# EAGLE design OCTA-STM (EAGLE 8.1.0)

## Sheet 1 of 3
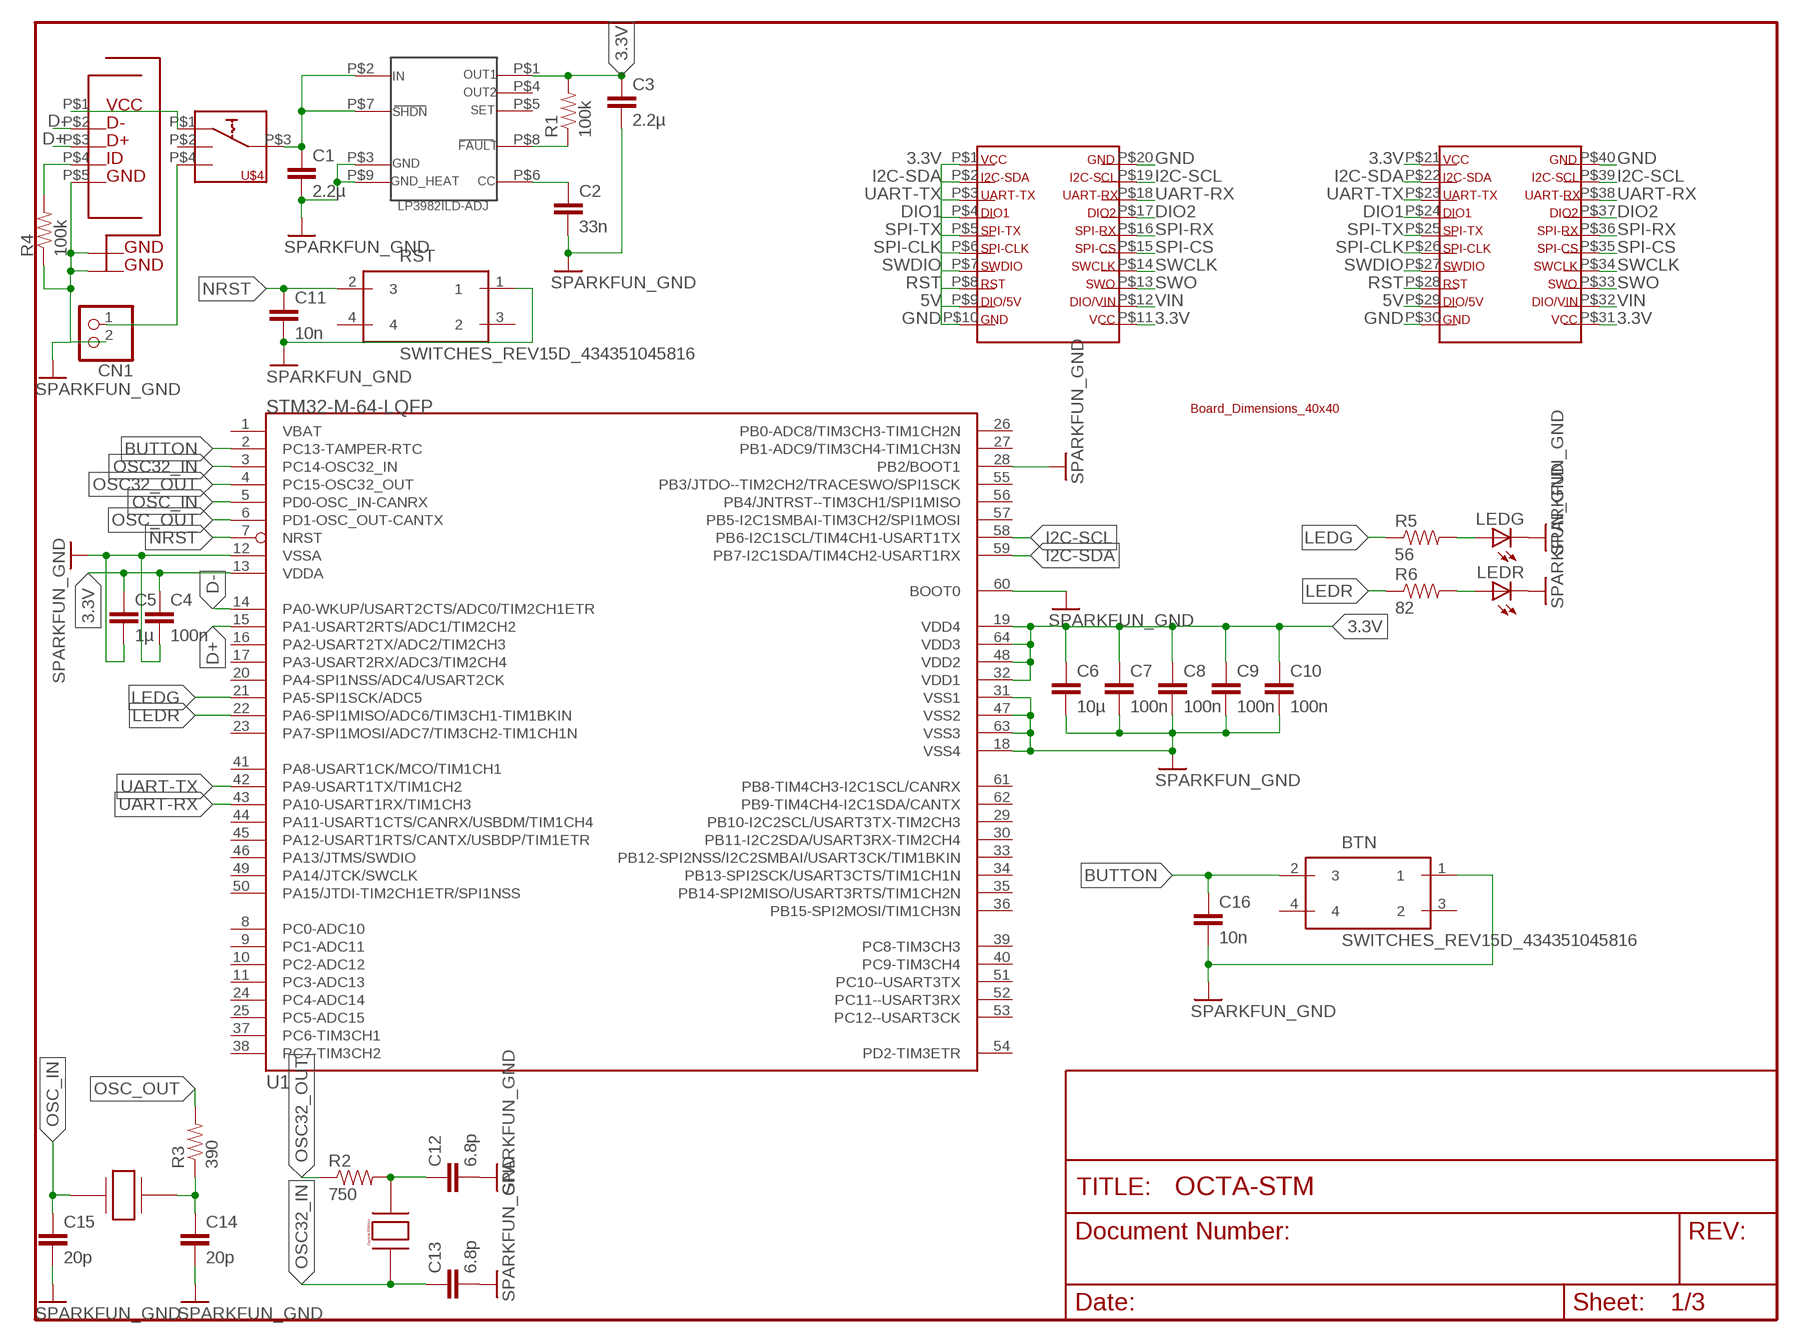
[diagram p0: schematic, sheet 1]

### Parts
8MHZ  OCTA-CORE_CRYSTAL-48MHZ  [OCTA-CORE_CRYSTAL-48MHZ]
BTN  SWITCHES_REV15D_434351045816  [SWITCHES_REV15D_434351045816]
C1  2.2µ  SPARKFUN_CAP0603-CAP  [SPARKFUN_0603-CAP]
C2  33n  SPARKFUN_CAP0603-CAP  [SPARKFUN_0603-CAP]
C3  2.2µ  SPARKFUN_CAP0603-CAP  [SPARKFUN_0603-CAP]
C4  100n  SPARKFUN_CAP0603-CAP  [SPARKFUN_0603-CAP]
C5  1µ  SPARKFUN_CAP0603-CAP  [SPARKFUN_0603-CAP]
C6  10µ  SPARKFUN_CAP0603-CAP  [SPARKFUN_0603-CAP]
C7  100n  SPARKFUN_CAP0603-CAP  [SPARKFUN_0603-CAP]
C8  100n  SPARKFUN_CAP0603-CAP  [SPARKFUN_0603-CAP]
C9  100n  SPARKFUN_CAP0603-CAP  [SPARKFUN_0603-CAP]
C10  100n  SPARKFUN_CAP0603-CAP  [SPARKFUN_0603-CAP]
C11  10n  SPARKFUN_CAP0603-CAP  [SPARKFUN_0603-CAP]
C12  6.8p  SPARKFUN_CAP0603-CAP  [SPARKFUN_0603-CAP]
C13  6.8p  SPARKFUN_CAP0603-CAP  [SPARKFUN_0603-CAP]
C14  20p  SPARKFUN_CAP0603-CAP  [SPARKFUN_0603-CAP]
C15  20p  SPARKFUN_CAP0603-CAP  [SPARKFUN_0603-CAP]
C16  10n  SPARKFUN_CAP0603-CAP  [SPARKFUN_0603-CAP]
CN1  ADAFRUIT_JST_2PIN-SMT-RA  [ADAFRUIT_JST-PH-2-SMT-RA]
LEDG  LED_LEDCHIP-LED0805  [LED_CHIP-LED0805]
LEDR  LED_LEDCHIP-LED0805  [LED_CHIP-LED0805]
R1  100k  SPARKFUN_RESISTOR0603-RES  [SPARKFUN_0603-RES]
R2  750  SPARKFUN_RESISTOR0603-RES  [SPARKFUN_0603-RES]
R3  390  SPARKFUN_RESISTOR0603-RES  [SPARKFUN_0603-RES]
R4  100k  SPARKFUN_RESISTOR0603-RES  [SPARKFUN_0603-RES]
R5  56  SPARKFUN_RESISTOR0603-RES  [SPARKFUN_0603-RES]
R6  82  SPARKFUN_RESISTOR0603-RES  [SPARKFUN_0603-RES]
RST  SWITCHES_REV15D_434351045816  [SWITCHES_REV15D_434351045816]
U1  STM32-M-64-LQFP  [LQFP64]
U$1  OCTA-CORE_MCIRO-USB2  [OCTA-CORE_MICRO-USB2]
U$2  BOARD-DIMENSIONS-40X40  [BOARD-DIMENSIONS-40X40]
U$3  DRAGAN-PERSONAL_TI-3.3V-REGULATOR  [DRAGAN-PERSONAL_TI-3.3V-REGULATOR]
U$4  OCTA-CORE_SP3T  [OCTA-CORE_SP3T]
U$5  DRAGAN-PERSONAL_CRYSTAL_32MHZ  [DRAGAN-PERSONAL_CRYSTAL_32MHZ]

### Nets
3.3V: C3.1 C4.1 C5.1 C6.1 C7.1 C8.1 C9.1 C10.1 R1.2 U1.13(VDDA) U1.19(VDD4) U1.32(VDD1) U1.48(VDD2) U1.64(VDD3) U$2.P$1 U$2.P$11 U$2.P$21 U$2.P$31 U$3.P$1 ; also sheet 2,3
5V: U$2.P$9 U$2.P$29
BUTTON: BTN.2 C16.1 U1.2(PC13-TAMPER-RTC)
D+: U1.15(PA1-USART2RTS/ADC1/TIM2CH2) U$1.P$3
D-: U1.14(PA0-WKUP/USART2CTS/ADC0/TIM2CH1ETR) U$1.P$2
DIO1: U$2.P$4 U$2.P$24
DIO2: U$2.P$17 U$2.P$37
GND: BTN.1 C1.2 C2.2 C3.2 C4.2 C5.2 C6.2 C7.2 C8.2 C9.2 C10.2 C11.2 C12.2 C13.2 C14.2 C15.2 C16.2 CN1.2 LEDG.C LEDR.C R4.1 RST.1 U1.12(VSSA) U1.18(VSS4) U1.28(PB2/BOOT1) U1.31(VSS1) U1.47(VSS2) U1.60(BOOT0) U1.63(VSS3) U$1.P$5 U$1.P$6 U$1.P$7 U$1.P$8 U$1.P$9 U$1.P$10 U$1.P$11 U$1.P$12 U$1.P$13 U$2.P$10 U$2.P$20 U$2.P$30 U$2.P$40 U$3.P$3 U$3.P$9 ; supply symbol labelled SPARKFUN_GND ; also sheet 2,3
I2C-SCL: U1.58(PB6-I2C1SCL/TIM4CH1-USART1TX) U$2.P$19 U$2.P$39 ; also sheet 2,3
I2C-SDA: U1.59(PB7-I2C1SDA/TIM4CH2-USART1RX) U$2.P$2 U$2.P$22 ; also sheet 2,3
LEDG: R5.1 U1.21(PA5-SPI1SCK/ADC5)
LEDR: R6.1 U1.22(PA6-SPI1MISO/ADC6/TIM3CH1-TIM1BKIN)
N$1: LEDG.A R5.2
N$2: CN1.1 U$4.P$4
N$3: U$1.P$1 U$4.P$1
N$4: C1.1 U$3.P$2 U$3.P$7 U$4.P$3
N$5: C2.1 U$3.P$6
N$6: C12.1 R2.2 U$5.P$2
N$7: R1.1 U$3.P$8
N$8: R4.2 U$1.P$4
N$9: 8MHZ.P$3 C14.1 R3.1
N$10: LEDR.A R6.2
NRST: C11.1 RST.2 U1.7(NRST)
OSC32_IN: C13.1 U1.3(PC14-OSC32_IN) U$5.P$3
OSC32_OUT: R2.1 U1.4(PC15-OSC32_OUT)
OSC_IN: 8MHZ.P$1 C15.1 U1.5(PD0-OSC_IN-CANRX)
OSC_OUT: R3.2 U1.6(PD1-OSC_OUT-CANTX)
RST: U$2.P$8 U$2.P$28
SPI-CLK: U$2.P$6 U$2.P$26
SPI-CS: U$2.P$15 U$2.P$35
SPI-RX: U$2.P$16 U$2.P$36
SPI-TX: U$2.P$5 U$2.P$25
SWCLK: U$2.P$14 U$2.P$34
SWDIO: U$2.P$7 U$2.P$27
SWO: U$2.P$13 U$2.P$33
UART-RX: U1.43(PA10-USART1RX/TIM1CH3) U$2.P$18 U$2.P$38
UART-TX: U1.42(PA9-USART1TX/TIM1CH2) U$2.P$3 U$2.P$23
VIN: U$2.P$12 U$2.P$32
Unconnected: 8MHZ.P$2 8MHZ.P$4 BTN.3 BTN.4 RST.3 RST.4 U1.1(VBAT) U1.8(PC0-ADC10) U1.9(PC1-ADC11) U1.10(PC2-ADC12) U1.11(PC3-ADC13) U1.16(PA2-USART2TX/ADC2/TIM2CH3) U1.17(PA3-USART2RX/ADC3/TIM2CH4) U1.20(PA4-SPI1NSS/ADC4/USART2CK) U1.23(PA7-SPI1MOSI/ADC7/TIM3CH2-TIM1CH1N) U1.24(PC4-ADC14) U1.25(PC5-ADC15) U1.26(PB0-ADC8/TIM3CH3-TIM1CH2N) U1.27(PB1-ADC9/TIM3CH4-TIM1CH3N) U1.29(PB10-I2C2SCL/USART3TX-TIM2CH3) U1.30(PB11-I2C2SDA/USART3RX-TIM2CH4) U1.33(PB12-SPI2NSS/I2C2SMBAI/USART3CK/TIM1BKIN) U1.34(PB13-SPI2SCK/USART3CTS/TIM1CH1N) U1.35(PB14-SPI2MISO/USART3RTS/TIM1CH2N) U1.36(PB15-SPI2MOSI/TIM1CH3N) U1.37(PC6-TIM3CH1) U1.38(PC7-TIM3CH2) U1.39(PC8-TIM3CH3) U1.40(PC9-TIM3CH4) U1.41(PA8-USART1CK/MCO/TIM1CH1) U1.44(PA11-USART1CTS/CANRX/USBDM/TIM1CH4) U1.45(PA12-USART1RTS/CANTX/USBDP/TIM1ETR) U1.46(PA13/JTMS/SWDIO) U1.49(PA14/JTCK/SWCLK) U1.50(PA15/JTDI-TIM2CH1ETR/SPI1NSS) U1.51(PC10--USART3TX) U1.52(PC11--USART3RX) U1.53(PC12--USART3CK) U1.54(PD2-TIM3ETR) U1.55(PB3/JTDO--TIM2CH2/TRACESWO/SPI1SCK) U1.56(PB4/JNTRST--TIM3CH1/SPI1MISO) U1.57(PB5-I2C1SMBAI-TIM3CH2/SPI1MOSI) U1.61(PB8-TIM4CH3-I2C1SCL/CANRX) U1.62(PB9-TIM4CH4-I2C1SDA/CANTX) U$3.P$4 U$3.P$5 U$4.P$2

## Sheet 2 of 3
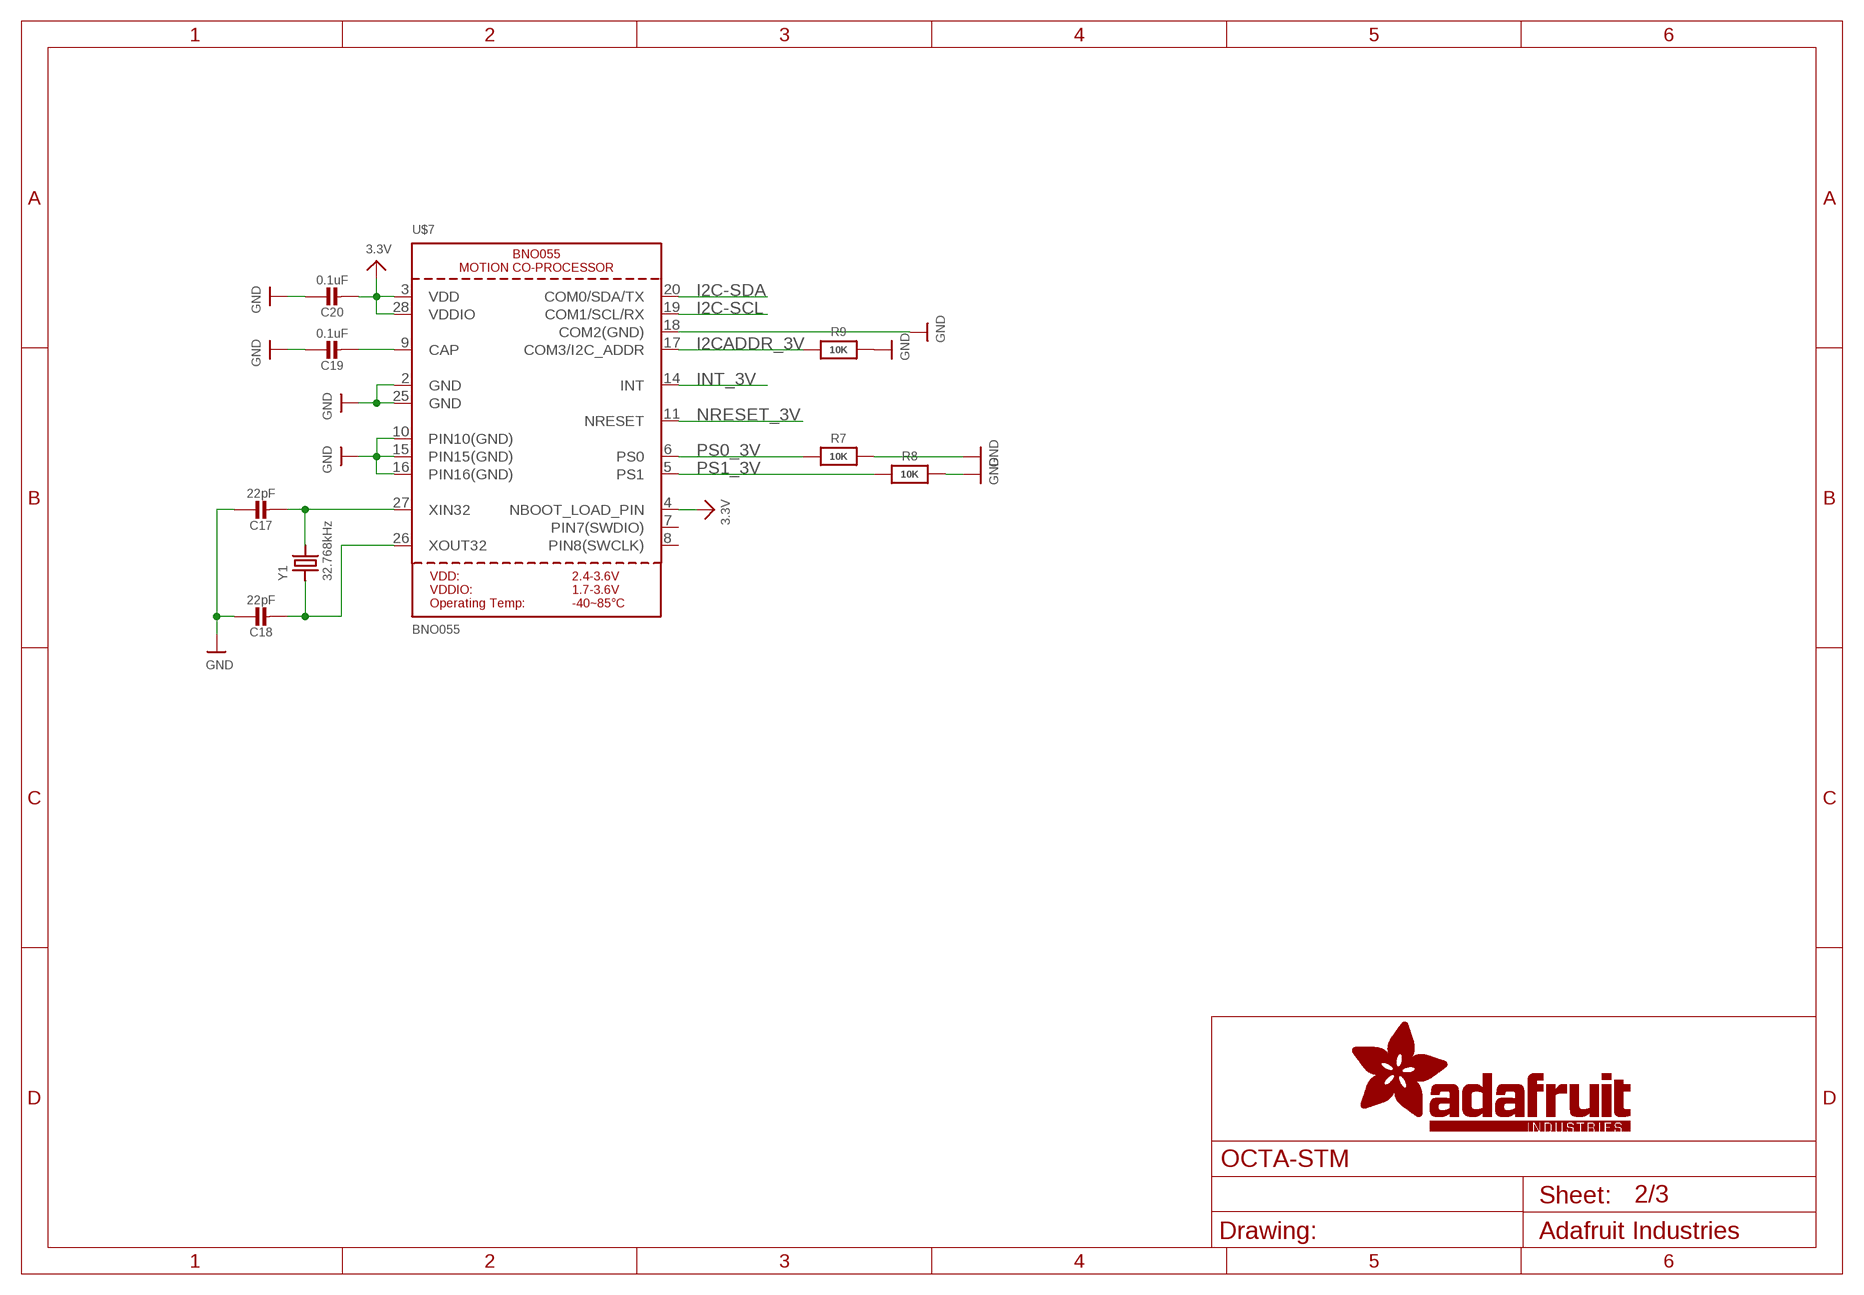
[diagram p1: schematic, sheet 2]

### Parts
C17  22pF  CAP_CERAMIC0805-NOOUTLINE  [0805-NO]
C18  22pF  CAP_CERAMIC0805-NOOUTLINE  [0805-NO]
C19  0.1uF  CAP_CERAMIC0805-NOOUTLINE  [0805-NO]
C20  0.1uF  CAP_CERAMIC0805_10MGAP  [0805_10MGAP]
R7  10K  RESISTOR0805_NOOUTLINE  [0805-NO]
R8  10K  RESISTOR0805_NOOUTLINE  [0805-NO]
R9  10K  RESISTOR0805_NOOUTLINE  [0805-NO]
U$7  BNO055  [BNO055]
Y1  32.768kHz  CRYSTAL8.0X3.8  [CRYSTAL_8X3.8]

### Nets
3.3V: C20.2 U$7.3(VDD) U$7.4(NBOOT_LOAD_PIN) U$7.28(VDDIO) ; also sheet 1,3
GND: C17.1 C18.1 C19.1 C20.1 R7.2 R8.2 R9.2 U$7.2(GND) U$7.10(PIN10(GND)) U$7.15(PIN15(GND)) U$7.16(PIN16(GND)) U$7.18(COM2(GND)) U$7.25(GND) ; also sheet 1,3
I2C-SCL: U$7.19(COM1/SCL/RX) ; also sheet 1,3
I2C-SDA: U$7.20(COM0/SDA/TX) ; also sheet 1,3
I2CADDR_3V: R9.1 U$7.17(COM3/I2C_ADDR)
INT_3V: U$7.14(INT)
N$11: C17.2 U$7.27(XIN32) Y1.P$4
N$12: C18.2 U$7.26(XOUT32) Y1.P$1
N$13: C19.2 U$7.9(CAP)
NRESET_3V: U$7.11(NRESET)
PS0_3V: R7.1 U$7.6(PS0)
PS1_3V: R8.1 U$7.5(PS1)
Unconnected: U$7.7(PIN7(SWDIO)) U$7.8(PIN8(SWCLK))

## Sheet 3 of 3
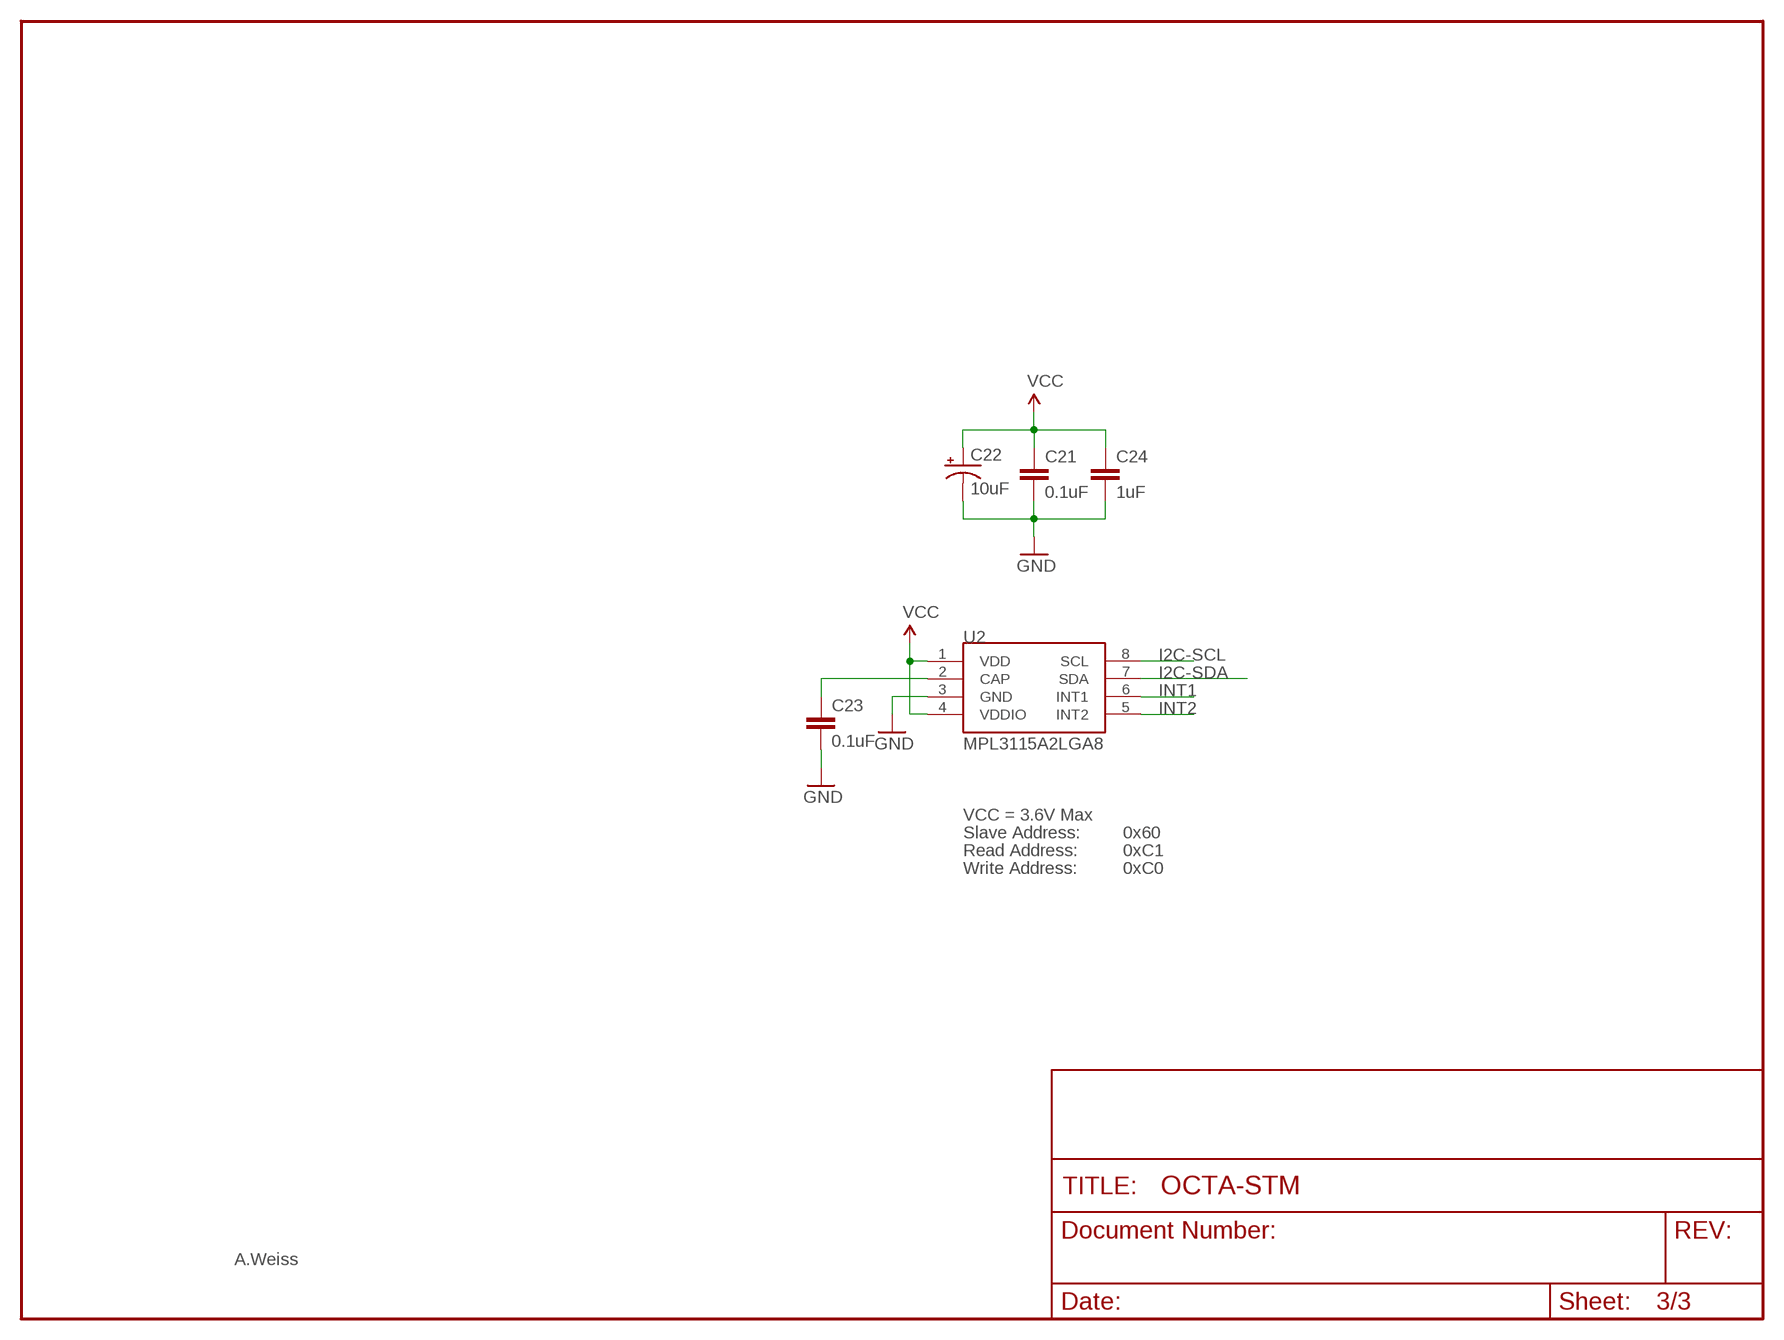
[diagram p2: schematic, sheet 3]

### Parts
C21  0.1uF  CAP0402-CAP  [0402-CAP]
C22  10uF  CAP_POL1206  [EIA3216]
C23  0.1uF  CAP0402-CAP  [0402-CAP]
C24  1uF  CAP0402-CAP  [0402-CAP]
U2  MPL3115A2LGA8  [LGA8]

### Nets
3.3V: C21.1 C22.A(+) C24.1 U2.1(VDD) U2.4(VDDIO) ; supply symbol labelled VCC ; also sheet 1,2
GND: C21.2 C22.C(-) C23.2 C24.2 U2.3(GND) ; also sheet 1,2
I2C-SCL: U2.8(SCL) ; also sheet 1,2
I2C-SDA: U2.7(SDA) ; also sheet 1,2
INT1: U2.6(INT1)
INT2: U2.5(INT2)
N$14: C23.1 U2.2(CAP)

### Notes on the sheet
- VCC = 3.6V Max
- Slave Address: | 0x60
- Read Address: | 0xC1
- Write Address: | 0xC0
- A.Weiss

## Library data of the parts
8MHZ = OCTA-EZR_v1:OCTA-CORE_CRYSTAL-48MHZ
BTN RST = OCTA-EZR_v1:SWITCHES_REV15D_434351045816: WS-TUS-3.5x4.7 mm side push SMD Tact Switch, 4 pins
C1-C16 = OCTA-EZR_v1:SPARKFUN_CAP: Capacitor
C17-C20 = microbuilder:CAP_CERAMIC: Ceramic Capacitors
C21 C23 C24 = SparkFun:CAP: Capacitor
C22 = SparkFun:CAP_POL: Capacitor Polarized
CN1 = OCTA-EZR_v1:ADAFRUIT_JST_2PIN: JST 2-Pin Connectors of various flavors
LEDG LEDR = OCTA-EZR_v1:LED_LED: LED
R1-R6 = OCTA-EZR_v1:SPARKFUN_RESISTOR: Resistor
R7-R9 = microbuilder:RESISTOR: Resistors
U1 = pel_stm32:STM32-M-64-LQFP: STM32F103 Medium Density 64pin LQFP
U2 = SparkFun-Sensors:MPL3115A2: Altimeter/Pressure Sensor, I2C, 1.95V-3.6V supply, 50 to 110kPa
U$1 = OCTA-EZR_v1:OCTA-CORE_MCIRO-USB2: Micr MICRO USB TYPE B RCPT W/ REAR PEGS. Mouser: 649-10118194-0001LF
U$2 = OCTA-CORE:BOARD-DIMENSIONS-40X40
U$3 = OCTA-EZR_v1:DRAGAN-PERSONAL_TI-3.3V-REGULATOR
U$4 = OCTA-EZR_v1:OCTA-CORE_SP3T
U$5 = OCTA-EZR_v1:DRAGAN-PERSONAL_CRYSTAL_32MHZ
U$7 = microbuilder:BNO055: BNO055 - Motion Co-Processor
Y1 = microbuilder:CRYSTAL: Crystals

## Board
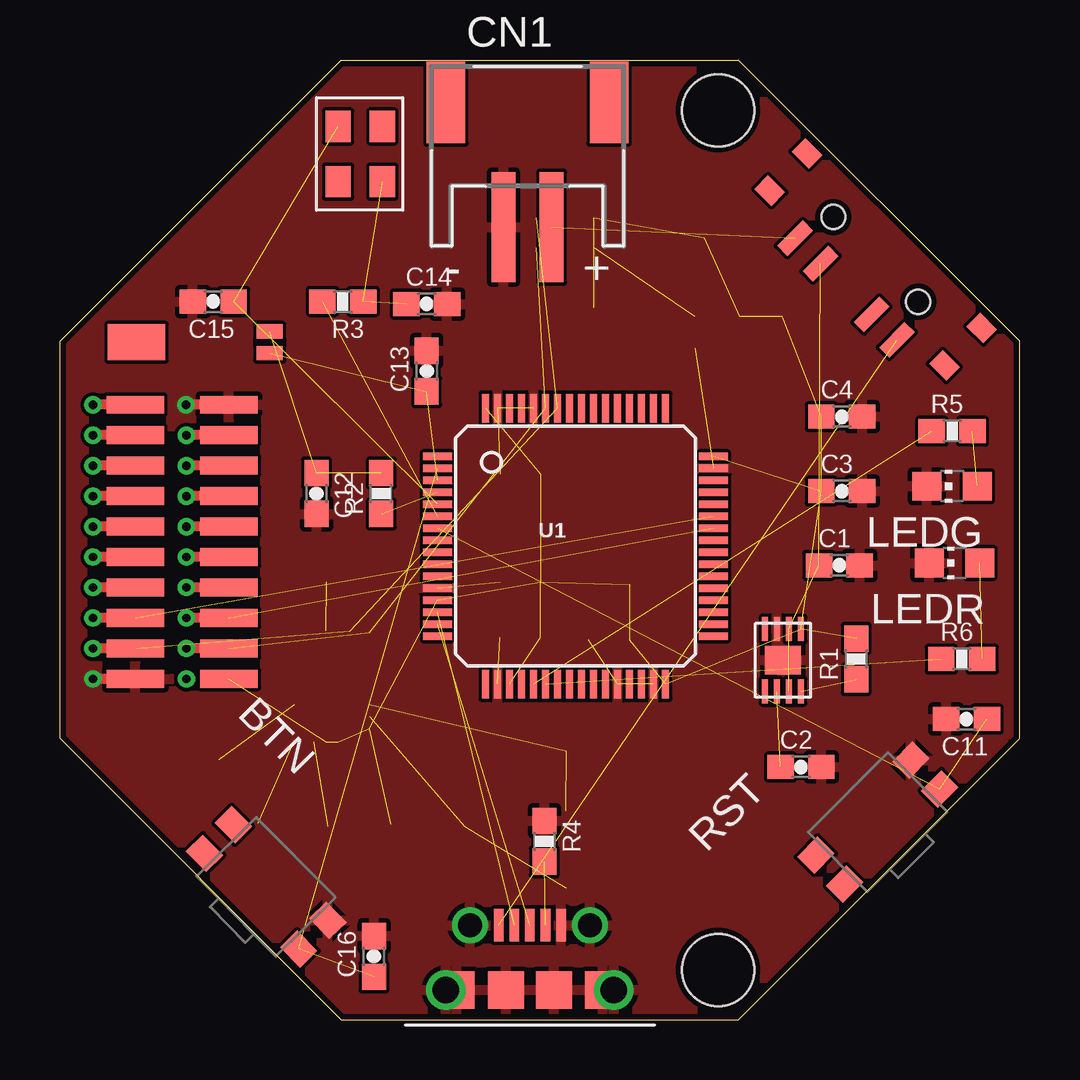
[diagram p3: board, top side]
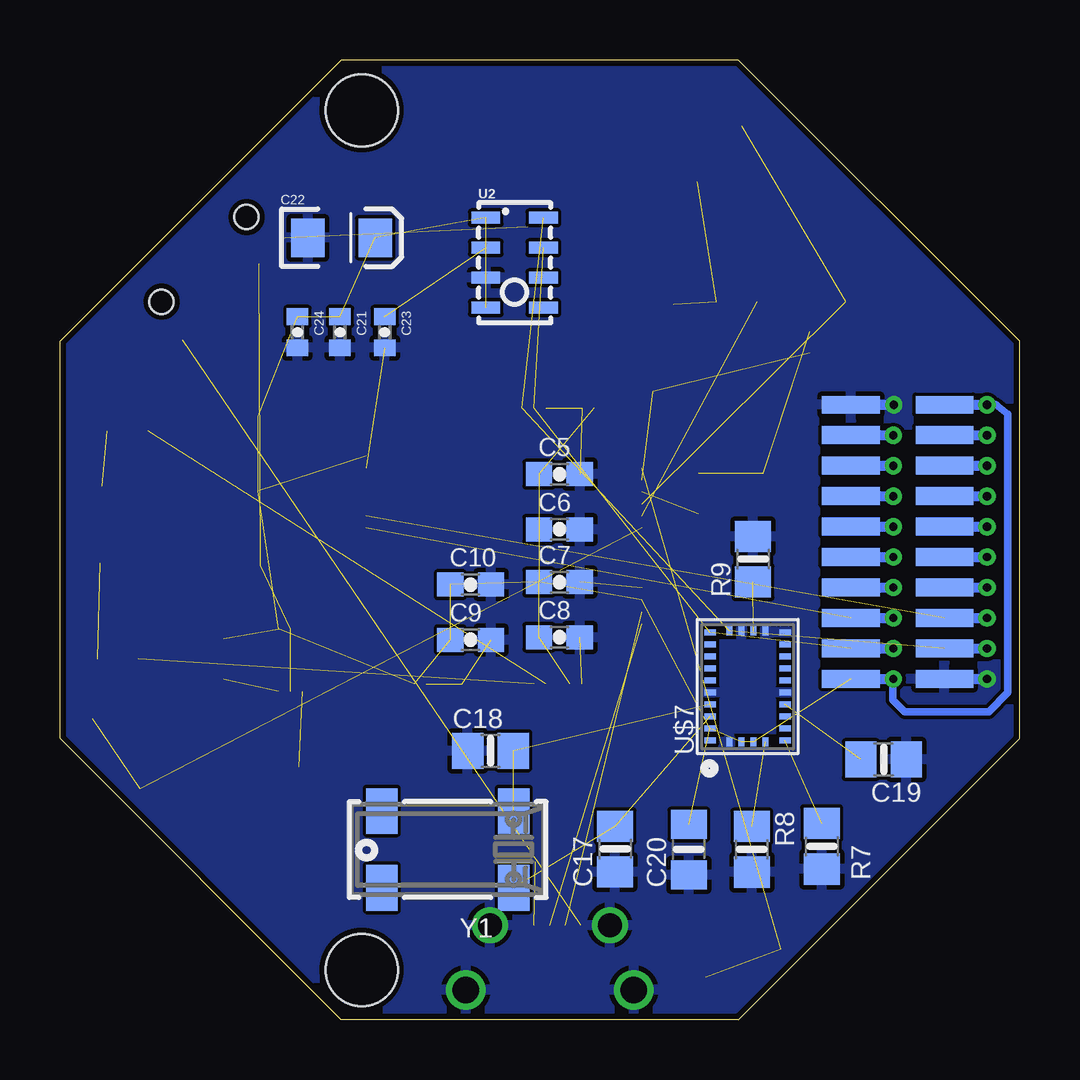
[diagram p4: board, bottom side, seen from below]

Size 40.01 x 40 mm. Coordinates in mm from the lower left corner, seen from the top.
Copper layers (1*16): Top 0.018mm / dielectric 1.55mm / Bottom 0.018mm
Design rules "eC_2Layer_PClass6_BaseCopperO18_eCDefault": minimum track width 0.15mm, minimum drill 0.35mm, track to track 0.15mm, track to pad 0.15mm, pad to pad 0.15mm, via to via 0.15mm, smd to smd 0mil, copper to edge 0.25mm, drill to drill 0.35mm, minimum pad ring 0.175mm, minimum via ring 0.125mm, stop-mask expansion 0mil, vias tented up to drill 0.45mm, thermal gap 0.2mm

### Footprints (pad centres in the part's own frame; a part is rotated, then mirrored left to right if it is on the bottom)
OCTA-CORE_CRYSTAL-48MHZ = smd 1.3 x 1.05: P$1 0,0; P$2 2.3,0; P$3 2.3,1.85; P$4 0,1.85
SWITCHES_REV15D_434351045816 = smd 1.2 x 1: 1 2.8,0.85; 2 2.8,-0.85; 3 -2.8,0.85; 4 -2.8,-0.85
SPARKFUN_0603-CAP = smd 1.1 x 1: 1 -0.85,0; 2 0.85,0
0805-NO = smd 1.3 x 1.5: 1 -0.95,0; 2 0.95,0
0805_10MGAP = smd 1.2 x 1.5: 1 -1.05,0; 2 1.05,0
0402-CAP = smd 0.7 x 0.9: 1 -0.65,0; 2 0.65,0
EIA3216 = smd 1.4 x 1.6: A 1.4,0; C -1.4,0
ADAFRUIT_JST-PH-2-SMT-RA = smd 1 x 4.6: 1 1,-3.7; 2 -1,-3.7 | smd 1.6 x 3.4: NC1 -3.4,1.5; NC2 3.4,1.5
LED_CHIP-LED0805 = smd 1.2 x 1.2: A 0,-1.05; C 0,1.05
SPARKFUN_0603-RES = smd 1.1 x 1: 1 -0.85,0; 2 0.85,0
LQFP64 = smd 1.2 x 0.3: 1 -5.75,3.75; 2 -5.75,3.25; 3 -5.75,2.75; 4 -5.75,2.25; 5 -5.75,1.75; 6 -5.75,1.25; 7 -5.75,0.75; 8 -5.75,0.25; 9 -5.75,-0.25; 10 -5.75,-0.75; 11 -5.75,-1.25; 12 -5.75,-1.75; 13 -5.75,-2.25; 14 -5.75,-2.75; 15 -5.75,-3.25; 16 -5.75,-3.75; 33 5.75,-3.75; 34 5.75,-3.25; 35 5.75,-2.75; 36 5.75,-2.25; 37 5.75,-1.75; 38 5.75,-1.25; 39 5.75,-0.75; 40 5.75,-0.25; 41 5.75,0.25; 42 5.75,0.75; 43 5.75,1.25; 44 5.75,1.75; 45 5.75,2.25; 46 5.75,2.75; 47 5.75,3.25; 48 5.75,3.75 | smd 0.3 x 1.2: 17 -3.75,-5.75; 18 -3.25,-5.75; 19 -2.75,-5.75; 20 -2.25,-5.75; 21 -1.75,-5.75; 22 -1.25,-5.75; 23 -0.75,-5.75; 24 -0.25,-5.75; 25 0.25,-5.75; 26 0.75,-5.75; 27 1.25,-5.75; 28 1.75,-5.75; 29 2.25,-5.75; 30 2.75,-5.75; 31 3.25,-5.75; 32 3.75,-5.75; 49 3.75,5.75; 50 3.25,5.75; 51 2.75,5.75; 52 2.25,5.75; 53 1.75,5.75; 54 1.25,5.75; 55 0.75,5.75; 56 0.25,5.75; 57 -0.25,5.75; 58 -0.75,5.75; 59 -1.25,5.75; 60 -1.75,5.75; 61 -2.25,5.75; 62 -2.75,5.75; 63 -3.25,5.75; 64 -3.75,5.75
LGA8 = smd 1.2 x 0.5: 1 -1.2,1.875; 2 -1.2,0.625; 3 -1.2,-0.625; 4 -1.2,-1.875; 5 1.2,-1.875; 6 1.2,-0.625; 7 1.2,0.625; 8 1.2,1.875
OCTA-CORE_MICRO-USB2 = smd 0.4 x 1.35: P$1 -1.3,0; P$2 -0.65,0; P$3 0,0; P$4 0.65,0; P$5 1.3,0 | drill 1 pad 1.5: P$6 -2.5,0; P$7 2.5,0 | smd 1.5 x 1.55: P$8 1,-2.7; P$9 -1,-2.7; P$10 -3.05,-2.7; P$11 3.05,-2.7 | drill 1.1 pad 1.6: P$12 -3.5,-2.7; P$13 3.5,-2.7
BOARD-DIMENSIONS-40X40 = smd 2.4 x 0.74: P$1 7.05,2.47; P$2 7.05,3.74; P$3 7.05,5.01; P$4 7.05,6.28; P$5 7.05,7.55; P$6 7.05,8.82; P$7 7.05,10.09; P$8 7.05,11.36; P$9 7.05,12.63; P$10 7.05,13.9; P$11 3.15,13.9; P$12 3.15,12.63; P$13 3.15,11.36; P$14 3.15,10.09; P$15 3.15,8.82; P$16 3.15,7.55; P$17 3.15,6.28; P$18 3.15,5.01; P$19 3.15,3.74; P$20 3.15,2.47 | smd 2.4 x 0.74 bottom: P$21 7.05,2.47; P$22 7.05,3.74; P$23 7.05,5.01; P$24 7.05,6.28; P$25 7.05,7.55; P$26 7.05,8.82; P$27 7.05,10.09; P$28 7.05,11.36; P$29 7.05,12.63; P$30 7.05,13.9; P$31 3.15,13.9; P$32 3.15,12.63; P$33 3.15,11.36; P$34 3.15,10.09; P$35 3.15,8.82; P$36 3.15,7.55; P$37 3.15,6.28; P$38 3.15,5.01; P$39 3.15,3.74; P$40 3.15,2.47 | hole 3: 27.44,26.17; 27.44,-9.66
DRAGAN-PERSONAL_TI-3.3V-REGULATOR = smd 0.25 x 1: P$1 0,-0.15; P$2 0.5,-0.15; P$3 1,-0.15; P$4 1.5,-0.15; P$5 1.5,2.45; P$6 1,2.45; P$7 0.5,2.45; P$8 0,2.45 | smd 1.5 x 1.2: P$9 0.75,1.15
OCTA-CORE_SP3T = smd 0.6 x 1.5: P$1 0,0; P$2 1.5,0; P$3 4.5,0; P$4 6,0 | smd 1 x 0.8: P$5 -2.15,-0.65; P$6 -2.15,-2.85; P$7 8.15,-0.65; P$8 8.15,-2.85 | hole 1: 0.5,-1.75; 5.5,-1.75
DRAGAN-PERSONAL_CRYSTAL_32MHZ = smd 2.4 x 1.5: P$1 0,0 | smd 1.1 x 0.6: P$2 5.55,0.45; P$3 5.55,-0.45
BNO055 = smd 0.25 x 0.475: 1 -2.25,1.562; 6 -2.25,-1.562; 7 -1.75,-1.562; 8 -1.25,-1.562; 9 -0.75,-1.562; 10 -0.25,-1.562; 11 0.25,-1.562; 12 0.75,-1.562; 13 1.25,-1.562; 14 1.75,-1.562; 15 2.25,-1.562; 20 2.25,1.562; 21 1.75,1.562; 22 1.25,1.562; 23 0.75,1.562; 24 0.25,1.562; 25 -0.25,1.562; 26 -0.75,1.562; 27 -1.25,1.562; 28 -1.75,1.562 | smd 0.375 x 0.25: 2 -2.312,0.75; 3 -2.312,0.25; 4 -2.312,-0.25; 5 -2.312,-0.75; 16 2.312,-0.75; 17 2.312,-0.25; 18 2.312,0.25; 19 2.312,0.75
CRYSTAL_8X3.8 = smd 1.3 x 1.9: P$1 -2.75,-1.6; P$2 2.75,-1.6; P$3 2.75,1.6; P$4 -2.75,1.6

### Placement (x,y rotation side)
8MHZ  11.59,37.23 270 top
BTN  8.59,5.53 314.6 top
C1  32.49,18.93 0 top
C2  30.89,10.53 0 top
C3  32.59,22.03 0 top
C4  32.59,25.13 0 top
C5  19.19,22.73 0 bottom
C6  19.19,20.43 0 bottom
C7  19.19,18.23 0 bottom
C8  19.19,15.93 0 bottom
C9  22.89,15.83 0 bottom
C10  22.89,18.13 0 bottom
C11  37.79,12.53 180 top
C12  10.69,21.93 270 top
C13  15.29,27.03 90 top
C14  15.29,29.83 0 top
C15  6.39,29.93 180 top
C16  13.09,2.63 90 top
C17  16.87,7.11 90 bottom
C18  22.06,11.2 0 bottom
C19  5.68,10.84 180 bottom
C20  13.8,7.09 90 bottom
C21  28.34,28.65 270 bottom
C22  28.27,32.59 0 bottom
C23  26.47,28.65 270 bottom
C24  30.11,28.65 270 bottom
CN1  19.49,36.73 0 top
LEDG  37.19,22.23 90 top
LEDR  37.29,19.03 90 top
R1  33.19,15.03 90 top
R2  13.39,21.93 90 top
R3  11.79,29.93 180 top
R4  20.19,7.43 270 top
R5  37.19,24.53 0 top
R6  37.59,15.03 0 top
R7  8.25,7.22 270 bottom
R8  11.17,7.1 270 bottom
R9  11.12,19.19 90 bottom
RST  34.09,8.23 45 top
U1  21.49,19.73 0 top
U2  21.06,31.55 0 bottom
U$1  19.59,3.93 0 top
U$2  -0.01,11.73 0 top
U$3  30.89,16.13 180 top
U$4  34.89,28.33 135 top
U$5  3.19,28.23 0 top
U$7  11.35,13.88 90 bottom
Y1  23.85,7.09 180 bottom

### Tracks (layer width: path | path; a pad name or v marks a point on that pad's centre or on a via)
3.3V  (via drill 0.35 pad 0.72)  (25 unrouted)
  Top 0.406: U$2.P$31 v1.37,25.63
  Bottom 0.305: v1.37,25.63 0.99,25.63 0.49,25.23 0.49,13.63 1.29,12.83 4.79,12.83 5.29,13.33 5.29,14.18 v5.27,14.2
  Bottom 0.406: U$2.P$31 v1.37,25.63 | U$2.P$1 v5.27,14.2
5V  (via drill 0.35 pad 0.72)
  Top 0.406: U$2.P$29 v5.27,24.36
  Bottom 0.406: U$2.P$29 v5.27,24.36
BUTTON  (2 unrouted)
D+  (1 unrouted)
D-  (1 unrouted)
DIO1  (via drill 0.35 pad 0.72)
  Top 0.406: U$2.P$24 v5.27,18.01
  Bottom 0.406: U$2.P$24 v5.27,18.01
DIO2  (via drill 0.35 pad 0.72)
  Top 0.406: U$2.P$37 v1.37,18.01
  Bottom 0.406: U$2.P$37 v1.37,18.01
GND  (via drill 0.35 pad 0.72)  (7 unrouted)
  Top 0.406: U$2.P$40 v1.37,14.2 | U$2.P$30 v5.25,25.63
  Bottom 0.406: U$2.P$40 v1.37,14.2 | U$2.P$30 v5.25,25.63
  pour Top: 0.09,28.33 11.69,39.93 28.39,39.93 40.09,28.23 40.09,11.73 28.29,-0.07 11.69,-0.07 0.09,11.53
  pour Bottom: -0.01,28.43 -0.01,11.63 11.69,-0.07 28.29,-0.07 40.09,11.73 40.09,28.23 28.39,39.93 11.69,39.93 11.39,39.93 11.39,39.83
I2C-SCL  (via drill 0.35 pad 0.72)  (3 unrouted)
  Top 0.406: U$2.P$39 v1.37,15.47
  Bottom 0.406: U$2.P$39 v1.37,15.47
I2C-SDA  (via drill 0.35 pad 0.72)  (3 unrouted)
  Top 0.406: U$2.P$22 v5.27,15.47
  Bottom 0.406: U$2.P$22 v5.27,15.47
I2CADDR_3V  (1 unrouted)
LEDG  (1 unrouted)
LEDR  (1 unrouted)
N$1  (1 unrouted)
N$2  (1 unrouted)
N$3  (1 unrouted)
N$4  (3 unrouted)
N$5  (1 unrouted)
N$6  (2 unrouted)
N$7  (1 unrouted)
N$8  (1 unrouted)
N$9  (2 unrouted)
N$10  (1 unrouted)
N$11  (2 unrouted)
N$12  (2 unrouted)
N$13  (1 unrouted)
N$14  (1 unrouted)
NRST  (2 unrouted)
OSC32_IN  (2 unrouted)
OSC32_OUT  (1 unrouted)
OSC_IN  (2 unrouted)
OSC_OUT  (1 unrouted)
PS0_3V  (1 unrouted)
PS1_3V  (1 unrouted)
RST  (via drill 0.35 pad 0.72)
  Top 0.406: U$2.P$28 v5.27,23.09
  Bottom 0.406: U$2.P$28 v5.27,23.09
SPI-CLK  (via drill 0.35 pad 0.72)
  Top 0.406: U$2.P$26 v5.27,20.55
  Bottom 0.406: U$2.P$26 v5.27,20.55
SPI-CS  (via drill 0.35 pad 0.72)
  Top 0.406: U$2.P$35 v1.37,20.55
  Bottom 0.406: U$2.P$35 v1.37,20.55
SPI-RX  (via drill 0.35 pad 0.72)
  Top 0.406: U$2.P$36 v1.37,19.28
  Bottom 0.406: U$2.P$36 v1.37,19.28
SPI-TX  (via drill 0.35 pad 0.72)
  Top 0.406: U$2.P$25 v5.27,19.28
  Bottom 0.406: U$2.P$25 v5.27,19.28
SWCLK  (via drill 0.35 pad 0.72)
  Top 0.406: U$2.P$34 v1.37,21.82
  Bottom 0.406: U$2.P$34 v1.37,21.82
SWDIO  (via drill 0.35 pad 0.72)
  Top 0.406: U$2.P$27 v5.27,21.82
  Bottom 0.406: U$2.P$27 v5.27,21.82
SWO  (via drill 0.35 pad 0.72)
  Top 0.406: U$2.P$33 v1.37,23.09
  Bottom 0.406: U$2.P$33 v1.37,23.09
UART-RX  (via drill 0.35 pad 0.72)  (1 unrouted)
  Top 0.406: U$2.P$38 v1.37,16.74
  Bottom 0.406: U$2.P$38 v1.37,16.74
UART-TX  (via drill 0.35 pad 0.72)  (1 unrouted)
  Top 0.406: U$2.P$23 v5.27,16.74
  Bottom 0.406: U$2.P$23 v5.27,16.74
VIN  (via drill 0.35 pad 0.72)
  Top 0.406: U$2.P$32 v1.37,24.36
  Bottom 0.406: U$2.P$32 v1.37,24.36

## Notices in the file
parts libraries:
SparkFun: Licensing: CC v3.0 Share-Alike You are welcome to use this library for commercial purposes.
microbuilder: This work is placed in the public domain, and may be freely used for commercial and non-commercial work with the following conditions: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
